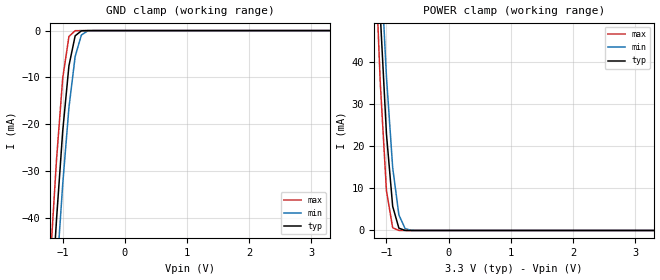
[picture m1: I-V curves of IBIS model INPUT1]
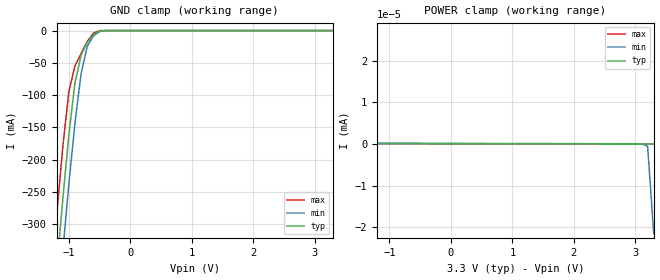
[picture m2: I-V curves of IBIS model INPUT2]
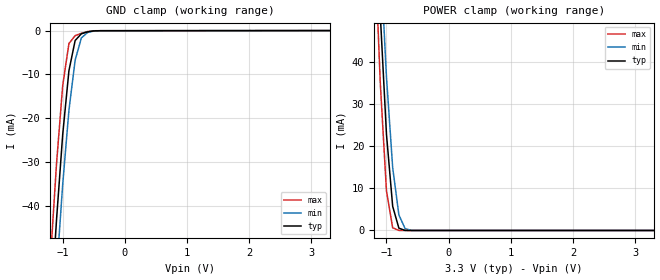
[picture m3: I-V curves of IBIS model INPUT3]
|   DIODES INCORPORATED
|   IBIS Model of PI6CG33402C
|   Product Family: 6CG
|   TQFN (ZH-32) Package
[IBIS Ver] 4.0
[Comment char] |_char
[File Name] pi6cg33402c_zh_reva.ibs
[File Rev] 1.0
[Source] File originated at Diodes Incorporated.
[Date] 04/02/2020
[Disclaimer] (C) Copyright DIODES INCORPORATED
   All rights reserved
  Diodes Incorporated hereby grants the user of
  this IBIS model a non-exclusive, nontransferable license to
  use this IBIS model under the following terms.
  This IBIS model is provided on an "AS IS" basis and Diodes
  makes absolutely no warranty with respect to the information
  contained herein. DIODES DISCLAIMS AND CUSTOMER WAIVES ALL
  WARRANTIES, EXPRESSED OR IMPLIED, INCLUDING WARRANTIES OF
  MERCHANTABILITY OR FITNESS FOR A PARTICULAR PURPOSE. The
  entire risk as to quality and performance is with the customer.
  Accordingly, in no event shall the company be liable for any
  damages, whether in contract or tort, including any lost
  profits or other incidental, consequential, exemplary, or
  punitive damages arising out of the use or application of the
  IBIS model provided in this package. Further, Diodes reserves
  the right to make changes without notice to any product herein
  to improve reliability, function, or design. Diodes does not
  convey any license under patent rights or any other intellectual
  property rights, including those of third parties.
  The user is granted this license only to use the IBIS model
  and is not granted rights to sell, load, rent, lease or license
  the IBIS model in whole or in part, or in modified form to anyone
  other than user. User may modify the IBIS model to suit its specific
  application but rights to derivative works and such modifications
  shall belong to Diodes.
  Diodes is not obligated to provide maintenance or support
  for the licensed IBIS model.
  Contact Diodes at ATTN: APPLICATION ENGINEERING / IBIS MODELS
  1545 Barber Ln. Milpitas, CA 95035
[Component] PI6CG33402C
[Manufacturer] Diodes Incorporated.
[Package]
| Variable   typ   min   max
R_pkg   0.03664ohm   0.02922ohm   0.04206ohm
L_pkg   0.78919nH   0.76828nH   0.81010nH
C_pkg   0.19084pF   0.17176pF   0.20992pF
[Pin]  signal_name   model_name   R_pin   L_pin   C_pin
1   GND   GND   0.04206   0.81010nH   0.20992pF
2   XTAL_IN/CLK   INPUT1   0.03778   0.79616nH   0.19720pF
3   XTAL_OUT   OUTPUT   0.03350   0.78222nH   0.18448pF
4   VDD_OSC   POWER   0.02922   0.76828nH   0.17176pF
5   VDD_REFOUT   POWER   0.02922   0.76828nH   0.17176pF
6   SADR/REFOUT   IO   0.03350   0.78222nH   0.18448pF
7   GND_REF   GND   0.03778   0.79616nH   0.19720pF
8   GND_DIG   GND   0.04206   0.81010nH   0.20992pF
9   VDD_DIG   POWER   0.04206   0.81010nH   0.20992pF
10   SCLK   INPUT2   0.03778   0.79616nH   0.19720pF
11   SDATA   IO_OS   0.03350   0.78222nH   0.18448pF
12   OE0#   INPUT3   0.02922   0.76828nH   0.17176pF
13   Q0+   HCSL_OUT   0.02922   0.76828nH   0.17176pF
14   Q0-   HCSL_OUT   0.03350   0.78222nH   0.18448pF
15   GND   GND   0.03778   0.79616nH   0.19720pF
16   VDDO   POWER   0.04206   0.81010nH   0.20992pF
17   OE1#   INPUT3   0.04206   0.81010nH   0.20992pF
18   Q1+   HCSL_OUT   0.03778   0.79616nH   0.19720pF
19   Q1-   HCSL_OUT   0.03350   0.78222nH   0.18448pF
20   GNDA   GND   0.02922   0.76828nH   0.17176pF
21   VDDA   POWER   0.02922   0.76828nH   0.17176pF
22   Q2+   HCSL_OUT   0.03350   0.78222nH   0.18448pF
23   Q2-   HCSL_OUT   0.03778   0.79616nH   0.19720pF
24   OE2#   INPUT3   0.04206   0.81010nH   0.20992pF
25   VDDO   POWER   0.04206   0.81010nH   0.20992pF
26   GND   GND   0.03778   0.79616nH   0.19720pF
27   Q3+   HCSL_OUT   0.03350   0.78222nH   0.18448pF
28   Q3-   HCSL_OUT   0.02922   0.76828nH   0.17176pF
29   OE3#   INPUT3   0.02922   0.76828nH   0.17176pF
30   GND   GND   0.03350   0.78222nH   0.18448pF
31   PD#   INPUT4   0.03778   0.79616nH   0.19720pF
32   SS_SEL_TRI   INPUT5   0.04206   0.81010nH   0.20992pF
| Models and submodels in the file (9): INPUT1 (Input), INPUT2 (Input), INPUT3 (Input), INPUT4 (Input), INPUT5 (Input), OUTPUT (Output), IO (I/O), IO_OS (I/O_open_sink), HCSL_OUT (Output)
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[Model] INPUT1
Model_type Input
Vinl = 825mV
Vinh = 2.75V
| variable   typ   min   max
C_comp   4.138pF   4.098pF   4.182pF
[Voltage Range]   3.3V   3.135V   3.465V
[GND Clamp Reference]   0.000V   0.000V   0.000V
[POWER Clamp Reference]   3.3V   3.135V   3.465V
[temperature range]   25   85   -40
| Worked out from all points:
|   GND clamp passes 1 mA (typ) near -0.79 V on its own axis
|   POWER clamp passes 1 mA (typ) near -0.81 V on its own axis
[GND Clamp]
| Voltage   I(typ)   I(min)   I(max)
-3.3V     -611mA     -617mA     -607mA
-1.2V     -62.2mA    -74.3mA    -49.3mA
-1.1V     -40.5mA    -52.6mA    -27.7mA
-1V       -21.5mA    -32.9mA    -10.2mA
-900mV    -7.54mA    -16.5mA    -1.27mA
-800mV    -1.13mA    -5.57mA    -24.2uA
-700mV    -53.2uA    -958uA     -202nA
-600mV    -1.35uA    -74.3uA    -1.53nA
3.3V      9.9pA      35.5pA     9.41pA
[POWER Clamp]   |Note: Vtable = Vcc - Voutput
| Voltage   I(typ)   I(min)   I(max)
-3.3V     1.02A      977mA      1.08A
-1.2V     86.3mA     99mA       71.7mA
-1.1V     51.3mA     65.5mA     35.1mA
-1V       22.8mA     36.4mA     9.39mA
-900mV    5.72mA     14.9mA     638uA
-800mV    544uA      3.68mA     8.25uA
-700mV    18.7uA     441uA      62.5nA
-600mV    428nA      26.6uA     460pA
3.3V      -9.9pA     -97pA      -9.41pA
[Model] INPUT2
Model_type Input
Vinl = 825mV
Vinh = 2.75V
| variable   typ   min   max
C_comp   2.377pF   2.375pF   2.379pF
[Voltage Range]   3.3V   3.135V   3.465V
[GND Clamp Reference]   0.000V   0.000V   0.000V
[POWER Clamp Reference]   3.3V   3.135V   3.465V
[temperature range]   25   85   -40
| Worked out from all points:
|   GND clamp passes 1 mA (typ) near -0.51 V on its own axis
|   POWER clamp passes 1 mA (typ) near -2.41 V on its own axis
[GND Clamp]
| Voltage   I(typ)   I(min)   I(max)
-3.3V     -3.1A      -3.15A     -3.08A
-1.3V     -486mA     -569mA     -402mA
-1.2V     -372mA     -455mA     -289mA
-1.1V     -263mA     -344mA     -182mA
-1V       -162mA     -238mA     -94.7mA
-900mV    -80.8mA    -143mA     -54.6mA
-800mV    -38mA      -66.3mA    -35.1mA
-700mV    -18.5mA    -24.4mA    -16.7mA
-600mV    -6.12mA    -8.27mA    -3.99mA
-500mV    -639uA     -1.47mA    -152uA
-400mV    -17.1uA    -85.9uA    -1.09uA
3.3V      65.7pA     151pA      64.9pA
[POWER Clamp]   |Note: Vtable = Vcc - Voutput
| Voltage   I(typ)   I(min)   I(max)
-3.3V     678mA      594mA      765mA
-2.2V     101nA      80.9nA     101nA
-2.1V     2.3nA      3.56nA     863pA
-2V       153pA      374pA      113pA
3.1V      4.4pA      39pA       7.18pA
3.2V      2.41pA     -514pA     5.21pA
3.3V      0A         -21.6nA    3.25pA
[Model] INPUT3
Model_type Input
Vinl = 825mV
Vinh = 2.75V
| variable   typ   min   max
C_comp   0.482pF   0.477pF   0.488pF
[Voltage Range]   3.3V   3.135V   3.465V
[GND Clamp Reference]   0.000V   0.000V   0.000V
[POWER Clamp Reference]   3.3V   3.135V   3.465V
[temperature range]   25   85   -40
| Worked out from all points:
|   GND clamp passes 1 mA (typ) near -0.72 V on its own axis
|   POWER clamp passes 1 mA (typ) near -0.81 V on its own axis
[GND Clamp]
| Voltage   I(typ)   I(min)   I(max)
-3.3V     -806mA     -784mA     -851mA
-1.2V     -65.6mA    -77.9mA    -52.7mA
-1.1V     -43.3mA    -55.5mA    -30.5mA
-1V       -23.7mA    -35.1mA    -12.5mA
-900mV    -9.15mA    -18.2mA    -2.93mA
-800mV    -2.24mA    -6.72mA    -1.13mA
-700mV    -702uA     -1.66mA    -594uA
-600mV    -266uA     -406uA     -185uA
-500mV    -41.5uA    -86.4uA    -13.4uA
3.3V      27.3uA     28.7uA     25.2uA
[POWER Clamp]   |Note: Vtable = Vcc - Voutput
| Voltage   I(typ)   I(min)   I(max)
-3.3V     1.02A      977mA      1.08A
-1.2V     86.3mA     99mA       71.7mA
-1.1V     51.3mA     65.5mA     35.1mA
-1V       22.8mA     36.4mA     9.39mA
-900mV    5.72mA     14.9mA     638uA
-800mV    544uA      3.68mA     8.25uA
-700mV    18.7uA     441uA      62.5nA
-600mV    428nA      26.6uA     460pA
3.3V      -9.9pA     -97pA      -9.41pA
